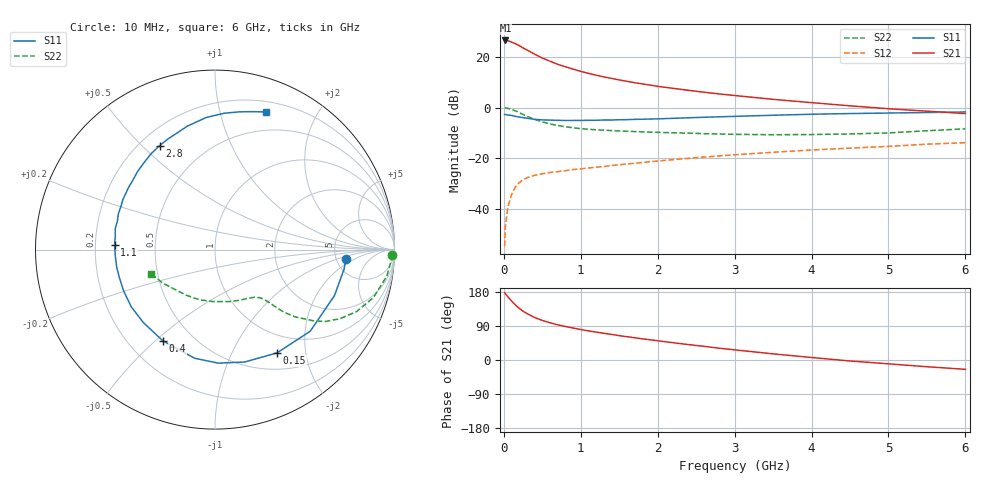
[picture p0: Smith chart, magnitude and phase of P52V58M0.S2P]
! SIEMENS Small Signal Semiconductors
! BFP183
! Si NPN RF Bipolar Junction Transistor in SOT143
! VCE = 2.5 V  IC = 8 mA
! Common Emitter S-Parameters:  March  1996
# GHz  S  MA  R  50
!  f  S11  S21  S12  S22
! GHz  MAG  ANG  MAG  ANG  MAG  ANG  MAG  ANG
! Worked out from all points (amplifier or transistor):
!   36 points, 10 MHz to 6 GHz, reference 50 ohm
!   highest |S21| = 26.6 dB at 20 MHz (marker M1)
!   |S21| within 3 dB of that: start of sweep to 251.5 MHz
!   unconditionally stable (mu >= 1): 1.262 GHz to 5.629 GHz
!   at 250 MHz: K = 0.28, MSG = 26.1 dB, |S12| = -28.6 dB
!   at 1.4 GHz: K = 1.05, MAG = 15.9 dB, |S12| = -23.0 dB
!   at 6 GHz: K = 0.96, MSG = 5.8 dB, |S12| = -13.9 dB
!   lowest NFmin = 1.30 dB at 450 MHz
!   S11 on the Smith chart (normalised r, x): 10 MHz: 6.07, -1.38; 150 MHz: 0.72, -1.52; 400 MHz: 0.34, -0.53; 1.1 GHz: 0.28, +0.02; 2.8 GHz: 0.28, +0.57; 6 GHz: 0.30, +1.40
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0.01  0.7294 -4.2  21.3 177.5  0.0018 83.4  0.9883 -1.7
0.02  0.7276 -8.5  21.34 175.3  0.0043 81.5  0.9837 -3.5
0.05  0.7132 -21.1  21.15 167.4  0.0103 83.3  0.9688 -8.8
0.1  0.6988 -40.6  19.78 155.9  0.019 70.4  0.9218 -16.9
0.15  0.6712 -59.0  18.43 145.3  0.0269 63.1  0.8606 -23.7
0.2  0.6478 -75.2  16.86 136.3  0.0326 56.9  0.7937 -29.1
0.25  0.6328 -88.4  15.15 128.8  0.037 51.9  0.7318 -33.2
0.3  0.6158 -100.7  13.81 122.7  0.0407 48.6  0.674 -36.0
0.4  0.5855 -119.7  11.45 112.1  0.0456 43.7  0.5835 -40.0
0.5  0.5697 -134.4  9.571 104.4  0.0489 40.1  0.5198 -42.2
0.6  0.5653 -145.5  8.285 98.2  0.0518 39.3  0.4748 -43.2
0.7  0.5588 -155.3  7.199 92.9  0.0539 38.3  0.4415 -43.9
0.9  0.5564 -169.8  5.776 84.4  0.0593 38.0  0.3981 -45.1
1.1  0.56 177.4  4.769 76.7  0.0637 38.5  0.3717 -46.6
1.5  0.5744 159.6  3.529 64.3  0.0738 39.3  0.3441 -50.5
1.8  0.5873 147.7  2.943 55.9  0.0816 39.9  0.3294 -54.9
2.2  0.6128 134.7  2.402 45.6  0.093 39.4  0.3168 -61.7
2.8  0.6565 118.0  1.863 31.1  0.1103 37.2  0.3002 -74.6
3.5  0.7049 102.6  1.456 16.2  0.1304 34.0  0.29 -92.3
4.5  0.7613 86.2  1.083 -2.6  0.1574 27.4  0.3003 -122.0
5.5  0.7979 74.4  0.849 -17.8  0.1884 21.1  0.3476 -147.8
6  0.8179 69.6  0.76 -24.6  0.2017 16.8  0.3797 -159.4
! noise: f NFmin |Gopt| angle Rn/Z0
0.45  1.3  0.17  43  0.21
0.9  1.35  0.21  115  0.2
1.8  2.05  0.33  -177  0.14
